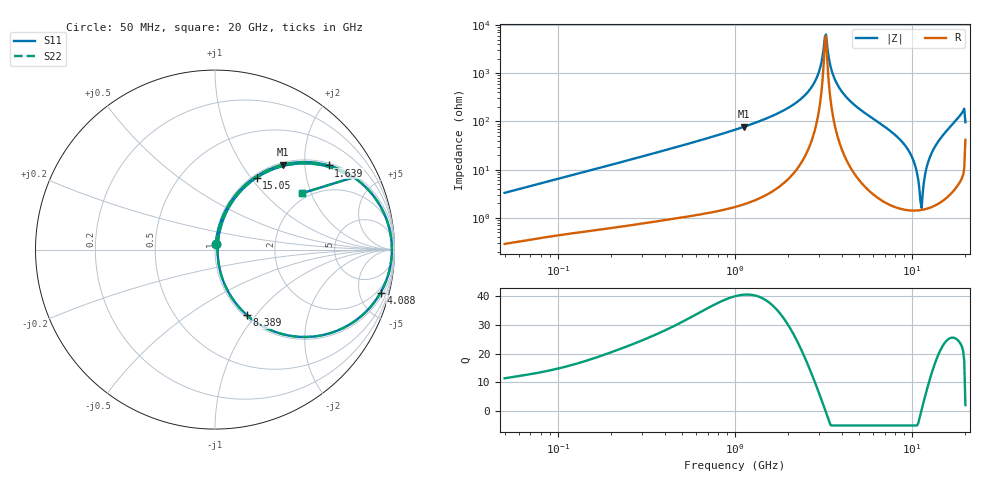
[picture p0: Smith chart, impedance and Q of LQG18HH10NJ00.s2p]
!Murata Part Number: LQG18HH10NJ00
!These Parameters are Measured in Series Mode Connection
!  o--[Z]--o
!Port1  Port2
!  o-------o
!Freq. Start=50[MHz] Stop=20[GHz], 401[Steps]
# Hz S RI R 50
!Freq.(Hz) S11(Real) S11(Imag) S21(Real) S21(Imag) S12(Real) S12(Imag) S22(Real) S22(Imag)
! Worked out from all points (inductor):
!   401 points, 50 MHz to 20 GHz, reference 50 ohm
!   read as one part in series: L = 10.4 nH near 51.52 MHz
!   highest Q = 40.5 at 1.127 GHz (marker M1), where L = 11 nH
!   self-resonance near 3.217 GHz
!   S11 on the Smith chart (normalised r, x): 50 MHz: 1.01, +0.07; 1.639 GHz: 1.07, +2.64; 4.088 GHz: 1.44, -7.58; 8.389 GHz: 1.03, -0.90; 15.05 GHz: 1.05, +1.07; 20 GHz: 1.83, +1.74
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5e7  0.00395 0.0327  0.996 -0.0327  0.996 -0.0327  0.00395 0.0327
1.364002e8  0.0124 0.0852  0.9876 -0.0852  0.9876 -0.0852  0.0124 0.0852
3.721004e8  0.059 0.218  0.941 -0.218  0.941 -0.218  0.059 0.218
1e9  0.3158 0.4525  0.6842 -0.4525  0.6842 -0.4525  0.3158 0.4525
1.127304e9  0.3802 0.4732  0.6198 -0.4732  0.6198 -0.4732  0.3802 0.4732
1.639343e9  0.6325 0.4687  0.3675 -0.4687  0.3675 -0.4687  0.6325 0.4687
2.245319e9  0.856 0.3311  0.144 -0.3311  0.144 -0.3311  0.856 0.3311
2.728004e9  0.9535 0.1742  0.0465 -0.1742  0.0465 -0.1742  0.9535 0.1742
2.98453e9  0.9779 0.087  0.0221 -0.087  0.0221 -0.087  0.9779 0.087
3.168813e9  0.985 0.0255  0.015 -0.0255  0.015 -0.0255  0.985 0.0255
3.265178e9  0.9857 -0.00588  0.0143 0.00588  0.0143 0.00588  0.9857 -0.00588
3.572216e9  0.9751 -0.101  0.0249 0.101  0.0249 0.101  0.9751 -0.101
4.087748e9  0.923 -0.2391  0.077 0.2391  0.077 0.2391  0.923 -0.2391
5.598765e9  0.6482 -0.4634  0.3518 0.4634  0.3518 0.4634  0.6482 -0.4634
7.442007e9  0.307 -0.4472  0.693 0.4472  0.693 0.4472  0.307 -0.4472
8.389408e9  0.1772 -0.3647  0.8228 0.3647  0.8228 0.3647  0.1772 -0.3647
1.004137e10  0.0422 -0.1644  0.9578 0.1644  0.9578 0.1644  0.0422 -0.1644
1.131968e10  0.0145 0.00671  0.9855 -0.00671  0.9855 -0.00671  0.0145 0.00671
1.257102e10  0.0447 0.1658  0.9553 -0.1658  0.9553 -0.1658  0.0447 0.1658
1.504638e10  0.2328 0.4015  0.7672 -0.4015  0.7672 -0.4015  0.2328 0.4015
1.912117e10  0.6847 0.4429  0.3153 -0.4429  0.3153 -0.4429  0.6847 0.4429
2e10  0.487 0.3146  0.513 -0.3146  0.513 -0.3146  0.487 0.3146
